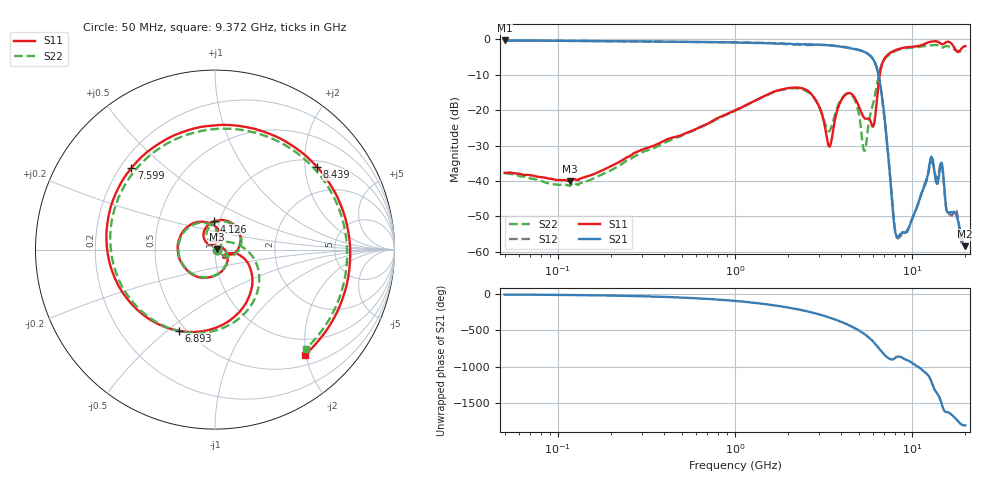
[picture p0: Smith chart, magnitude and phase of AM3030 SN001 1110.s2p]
# Hz S DB R 50
!freq MagS11 AngS11 MagS21 AngS21 MagS12 AngS12 MagS22 AngS22
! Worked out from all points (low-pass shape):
!   1601 points, 50 MHz to 20.05 GHz, reference 50 ohm
!   highest |S21| = -0.34 dB at 50 MHz (marker M1); lowest = -58.4 dB at 19.9 GHz (marker M2)
!   |S21| within 3 dB of the highest: start of sweep to 5.25 GHz
!   lowest |S11| = -40.2 dB at 117 MHz (marker M3), VSWR 1.02, Z = 51 + j0.162 ohm
!   |S11| at or under -10 dB: start of sweep to 6.581 GHz
!   |S22| runs from -41.4 to -1.6 dB; largest |S21 - S12| = 0.026
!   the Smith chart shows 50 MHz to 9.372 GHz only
!   S11 on the Smith chart (normalised r, x): 50 MHz: 1.03, -0.01; 4.126 GHz: 0.94, +0.30; 6.893 GHz: 0.46, -0.55; 7.599 GHz: 0.24, +0.39; 8.439 GHz: 1.16, +2.31; 9.372 GHz: 0.69, -1.98
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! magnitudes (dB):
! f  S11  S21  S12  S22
! 50 MHz  -37.7  -0.3  -0.4  -37.8
! 117 MHz  -40.2  -0.5  -0.5  -41.4
! 135.9 MHz  -39.2  -0.5  -0.5  -40.6
! 369.6 MHz  -29.5  -0.7  -0.7  -30.1
! 1.005 GHz  -20.0  -0.9  -0.9  -20.2
! 2.722 GHz  -15.6  -1.5  -1.6  -15.8
! 3.421 GHz  -30.3  -1.7  -1.7  -25.9
! 4.126 GHz  -16.1  -2.2  -2.2  -16.0
! 4.775 GHz  -16.7  -2.8  -2.8  -17.3
! 5.404 GHz  -22.3  -3.6  -3.6  -31.5
! 6.069 GHz  -24.4  -5.8  -5.8  -17.6
! 6.893 GHz  -6.1  -19.0  -19.6  -6.1
! 7.402 GHz  -4.1  -34.6  -34.4  -4.5
! 7.599 GHz  -3.7  -41.4  -40.8  -4.1
! 8.008 GHz  -3.1  -53.9  -53.3  -3.4
! 8.439 GHz  -2.7  -55.6  -56.0  -2.9
! 9.372 GHz  -2.3  -54.4  -54.0  -2.5
! 12.89 GHz  -0.7  -33.2  -34.8  -1.7
! 14.64 GHz  -1.3  -34.9  -34.9  -2.3
! 15.89 GHz  -0.7  -48.9  -49.2  -2.0
! 19.9 GHz  -2.0  -58.4  -58.1  -3.3
! 20.05 GHz  -1.9  -58.2  -57.9  -3.3
